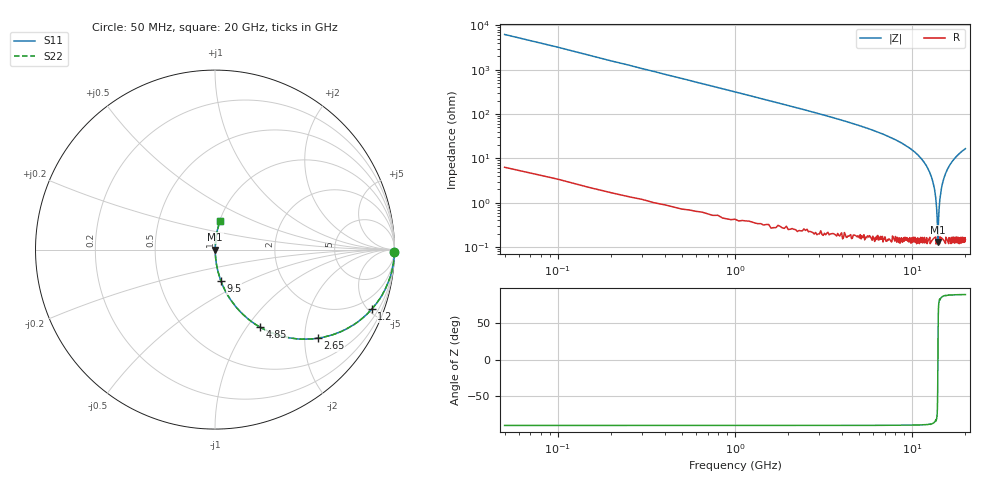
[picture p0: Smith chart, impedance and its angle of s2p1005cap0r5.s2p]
!	AVX	Thin	Film	Operation
!	Date:	March 2012
!	Description: Ultra-Miniature 01005 Size ACCU - P® Thin Film RF / Microwave Capacitor
!	Part Number:  C005YJ0R5ABSTR
!	Serial	Measurements
# MHZ S MA R 50
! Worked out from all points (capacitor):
!   400 points, 50 MHz to 20 GHz, reference 50 ohm
!   read as one part in series: C = 499 fF near 150 MHz
!   lowest |Z| = 130 mohm at 14 GHz (marker M1)
!   series resonance near 13.99 GHz, so ESL is about 260 pH
!   S11 on the Smith chart (normalised r, x): 50 MHz: open; 1.2 GHz: 1.01, -5.26; 2.65 GHz: 1.00, -2.32; 4.85 GHz: 1.00, -1.15; 9.5 GHz: 1.00, -0.36; 20 GHz: 1.00, +0.33
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50  1 -0.9  0.016 89.0  0.016 89.0  1 -0.9
150  0.999 -2.7  0.047 87.2  0.047 87.2  0.999 -2.7
400  0.992 -7.2  0.125 82.8  0.125 82.8  0.992 -7.2
750  0.973 -13.3  0.23 76.6  0.23 76.6  0.973 -13.3
1200  0.934 -20.8  0.355 69.1  0.355 69.1  0.934 -20.8
2650  0.756 -40.8  0.653 49.1  0.653 49.1  0.756 -40.8
3400  0.66 -48.6  0.75 41.3  0.75 41.3  0.66 -48.6
4850  0.499 -59.9  0.865 30.0  0.865 30.0  0.499 -59.9
6700  0.343 -69.7  0.938 20.1  0.938 20.1  0.343 -69.7
9500  0.177 -79.3  0.983 10.2  0.983 10.2  0.177 -79.3
10050  0.151 -80.8  0.987 8.7  0.987 8.7  0.151 -80.8
12350  0.057 -85.3  0.997 3.2  0.997 3.2  0.057 -85.3
13350  0.021 -84.9  0.998 1.2  0.998 1.2  0.021 -84.9
13750  0.007859 -79.0  0.999 0.4  0.999 0.4  0.007859 -79.0
14000  0.001506 17.9  0.999 -0.0  0.999 -0.0  0.001506 17.9
14100  0.003967 68.6  0.999 -0.2  0.999 -0.2  0.003967 68.6
14200  0.007058 77.9  0.999 -0.4  0.999 -0.4  0.007058 77.9
14350  0.012 82.3  0.998 -0.7  0.998 -0.7  0.012 82.3
14600  0.02 84.7  0.998 -1.1  0.998 -1.1  0.02 84.7
15400  0.044 85.6  0.998 -2.5  0.998 -2.5  0.044 85.6
16700  0.081 84.3  0.995 -4.6  0.995 -4.6  0.081 84.3
20000  0.164 80.1  0.985 -9.4  0.985 -9.4  0.164 80.1
